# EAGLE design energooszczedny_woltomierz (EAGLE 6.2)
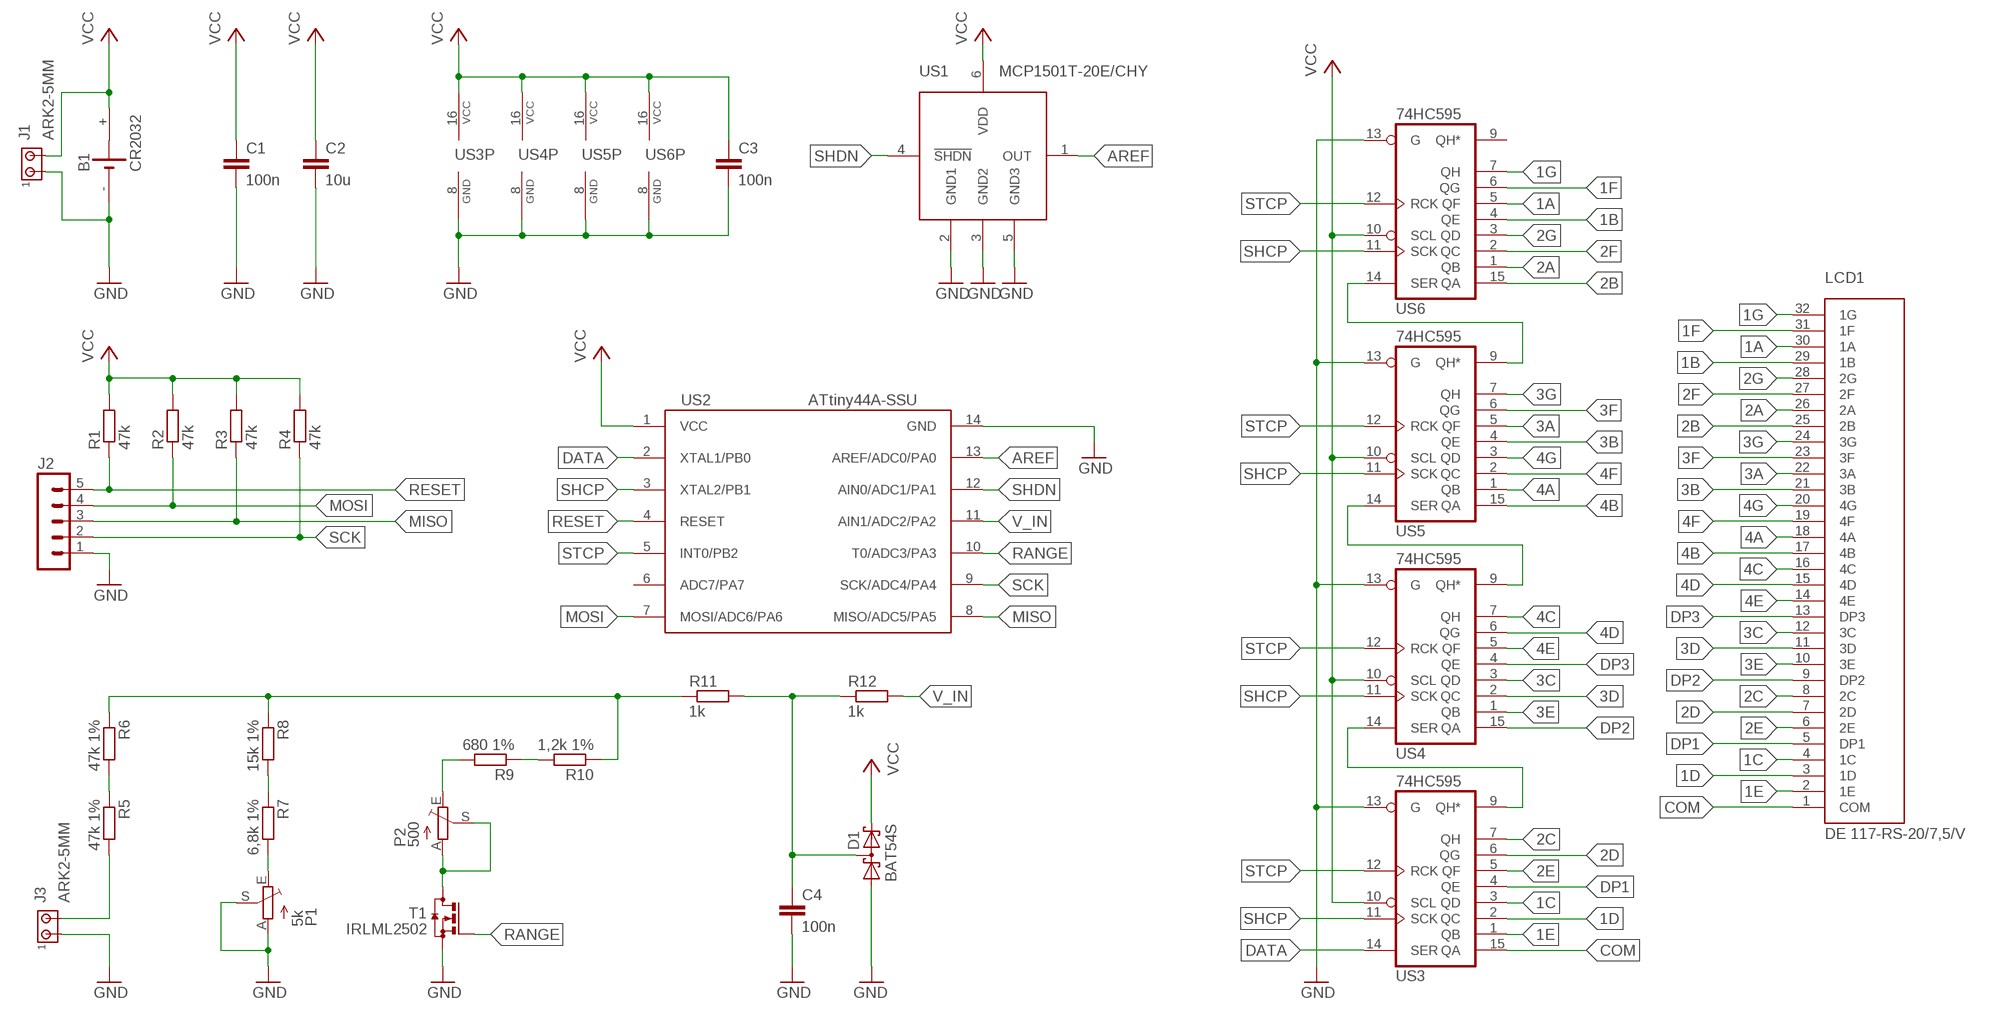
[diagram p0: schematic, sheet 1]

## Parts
B1  CR2032  BAT_20/16_XX  [BAT_CR2032]
C1  100n  C-EUC0805  [C0805]
C2  10u  C-EUC0805  [C0805]
C3  100n  C-EUC0805  [C0805]
C4  100n  C-EUC0805  [C0805]
D1  BAT54S  [SOT23]
J1  ARK2-5MM  [2PIN-5MM]
J2  MA05-1  [MA05-1]
J3  ARK2-5MM  [2PIN-5MM]
LCD1  DE 117-RS-20/7,5/V  LCD_DE117  [DE117]
P1  5k  TRIM_EU-CA6V  [CA6V]
P2  500  TRIM_EU-CA6V  [CA6V]
R1  47k  R-EU_R0805  [R0805]
R2  47k  R-EU_R0805  [R0805]
R3  47k  R-EU_R0805  [R0805]
R4  47k  R-EU_R0805  [R0805]
R5  47k 1%  R-EU_R0805  [R0805]
R6  47k 1%  R-EU_R0805  [R0805]
R7  6,8k 1%  R-EU_R0805  [R0805]
R8  15k 1%  R-EU_R0805  [R0805]
R9  680 1%  R-EU_R0805  [R0805]
R10  1,2k 1%  R-EU_R0805  [R0805]
R11  1k  R-EU_R0805  [R0805]
R12  1k  R-EU_R0805  [R0805]
T1  IRLML2502  BSS123  [SOT23]
US1  MCP1501T-20E/CHY  MCP1501  [SOT23-6]
US2  ATtiny44A-SSU  ATTINY24/44/84-SSU  [SOIC14]
US3  74HC595  74LS595D  [SO16]
US4  74HC595  74LS595D  [SO16]
US5  74HC595  74LS595D  [SO16]
US6  74HC595  74LS595D  [SO16]

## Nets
1A: LCD1.30(1A) US6.5(QF)
1B: LCD1.29(1B) US6.4(QE)
1C: LCD1.4(1C) US3.3(QD)
1D: LCD1.3(1D) US3.2(QC)
1E: LCD1.2(1E) US3.1(QB)
1F: LCD1.31(1F) US6.6(QG)
1G: LCD1.32(1G) US6.7(QH)
2A: LCD1.26(2A) US6.1(QB)
2B: LCD1.25(2B) US6.15(QA)
2C: LCD1.8(2C) US3.7(QH)
2D: LCD1.7(2D) US3.6(QG)
2E: LCD1.6(2E) US3.5(QF)
2F: LCD1.27(2F) US6.2(QC)
2G: LCD1.28(2G) US6.3(QD)
3A: LCD1.22(3A) US5.5(QF)
3B: LCD1.21(3B) US5.4(QE)
3C: LCD1.12(3C) US4.3(QD)
3D: LCD1.11(3D) US4.2(QC)
3E: LCD1.10(3E) US4.1(QB)
3F: LCD1.23(3F) US5.6(QG)
3G: LCD1.24(3G) US5.7(QH)
4A: LCD1.18(4A) US5.1(QB)
4B: LCD1.17(4B) US5.15(QA)
4C: LCD1.16(4C) US4.7(QH)
4D: LCD1.15(4D) US4.6(QG)
4E: LCD1.14(4E) US4.5(QF)
4F: LCD1.19(4F) US5.2(QC)
4G: LCD1.20(4G) US5.3(QD)
AREF: US1.1(OUT) US2.13(AREF/ADC0/PA0)
COM: LCD1.1(COM) US3.15(QA)
DATA: US2.2(XTAL1/PB0) US3.14(SER)
DP1: LCD1.5(DP1) US3.4(QE)
DP2: LCD1.9(DP2) US4.15(QA)
DP3: LCD1.13(DP3) US4.4(QE)
GND: B1.- C1.2 C2.2 C3.2 C4.2 D1.1(A1) J1.P$1 J2.1 J3.P$1 P1.A P1.S T1.2(S) US1.2(GND1) US1.3(GND2) US1.5(GND3) US2.14(GND) US3.8(GND) US3.13(G) US4.8(GND) US4.13(G) US5.8(GND) US5.13(G) US6.8(GND) US6.13(G)
MISO: J2.3 R3.1 US2.8(MISO/ADC5/PA5)
MOSI: J2.4 R2.1 US2.7(MOSI/ADC6/PA6)
N$1: J3.P$2 R5.2
N$2: R5.1 R6.2
N$3: R6.1 R8.1 R10.1 R11.1
N$4: C4.1 D1.3(C1A2) R11.2 R12.1
N$5: P2.A P2.S T1.3(D)
N$6: R7.1 R8.2
N$7: R9.1 R10.2
N$8: P1.E R7.2
N$9: P2.E R9.2
N$33: US3.9(QH*) US4.14(SER)
N$34: US4.9(QH*) US5.14(SER)
N$35: US5.9(QH*) US6.14(SER)
RANGE: T1.1(G) US2.10(T0/ADC3/PA3)
RESET: J2.5 R1.1 US2.4(RESET)
SCK: J2.2 R4.1 US2.9(SCK/ADC4/PA4)
SHCP: US2.3(XTAL2/PB1) US3.11(SCK) US4.11(SCK) US5.11(SCK) US6.11(SCK)
SHDN: US1.4(!SHDN) US2.12(AIN0/ADC1/PA1)
STCP: US2.5(INT0/PB2) US3.12(RCK) US4.12(RCK) US5.12(RCK) US6.12(RCK)
V_IN: R12.2 US2.11(AIN1/ADC2/PA2)
VCC: B1.+ C1.1 C2.1 C3.1 D1.2(C2) J1.P$2 R1.2 R2.2 R3.2 R4.2 US1.6(VDD) US2.1(VCC) US3.10(SCL) US3.16(VCC) US4.10(SCL) US4.16(VCC) US5.10(SCL) US5.16(VCC) US6.10(SCL) US6.16(VCC)
Unconnected: US2.6(ADC7/PA7) US6.9(QH*)

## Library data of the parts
B1 = inne_futrzak:BAT_20/16_XX
C1-C4 = rcl:C-EU: CAPACITOR, European symbol
D1 = diode:BAT54S: Schottky Diodes Pin connection corrected 2011-05-04 Source: Fairchild .. BAT54.pdf
J1 J3 = zlacza_futrzak:ARK2: ARK 2
J2 = zlacza_futrzak:MA05-1: PIN HEADER; OC_FARNELL: unknown; OC_NEWARK: unknown
LCD1 = inne_futrzak:LCD_DE117
P1 P2 = pot:TRIM_EU-: POTENTIOMETER
R1-R12 = rcl:R-EU_: RESISTOR, European symbol
T1 = transistor-small-signal:BSS123: N-CHANNEL MOS FET
US1 = scalaki_futrzak:MCP1501
US2 = scalaki_futrzak:ATTINY24/44/84
US3-US6 = scalaki_futrzak:74*595: 8-bit SHIFT REGISTER, output latch

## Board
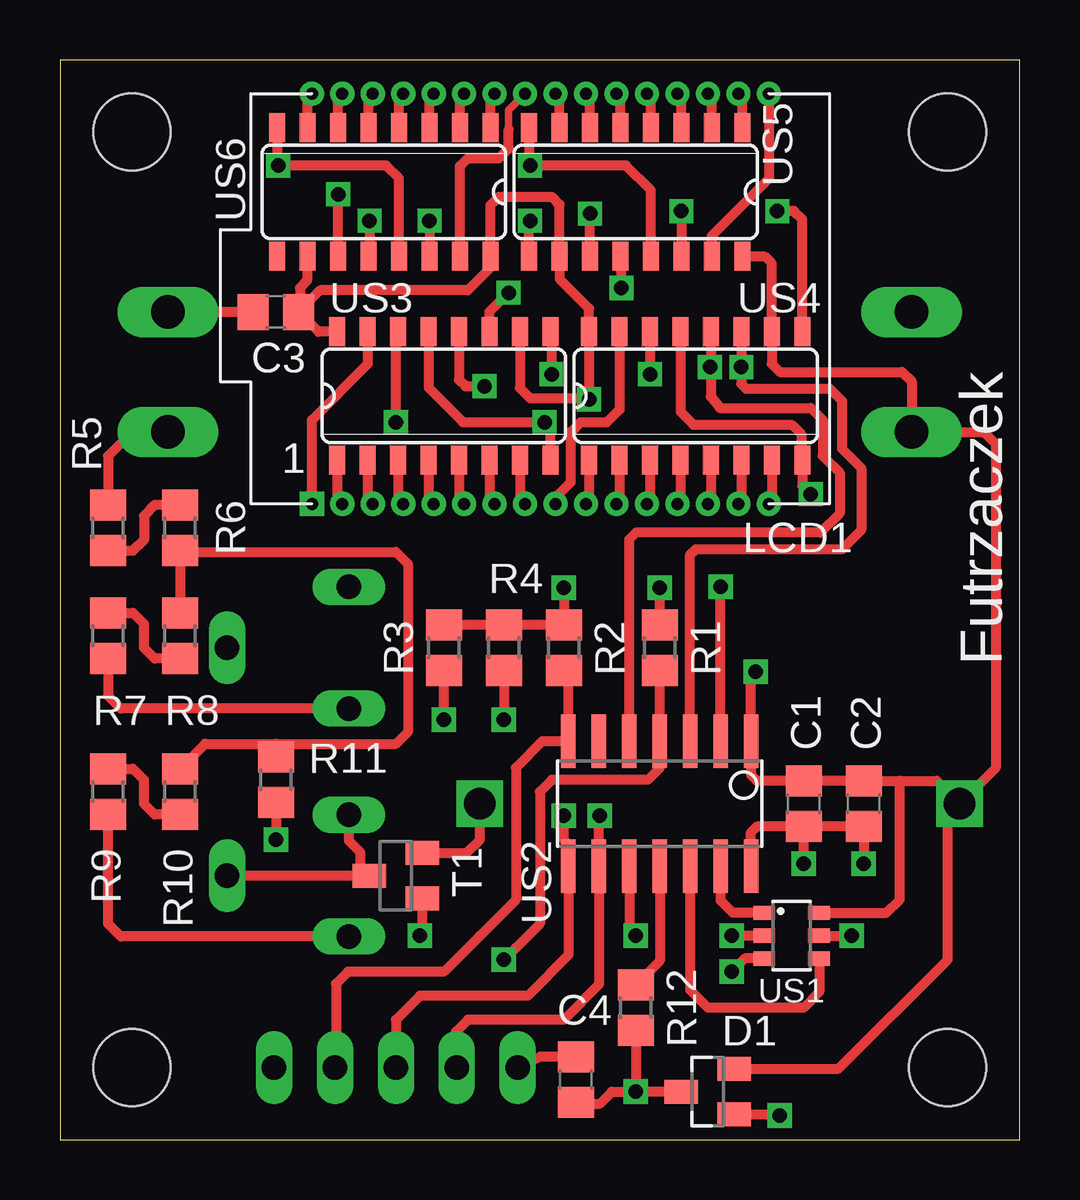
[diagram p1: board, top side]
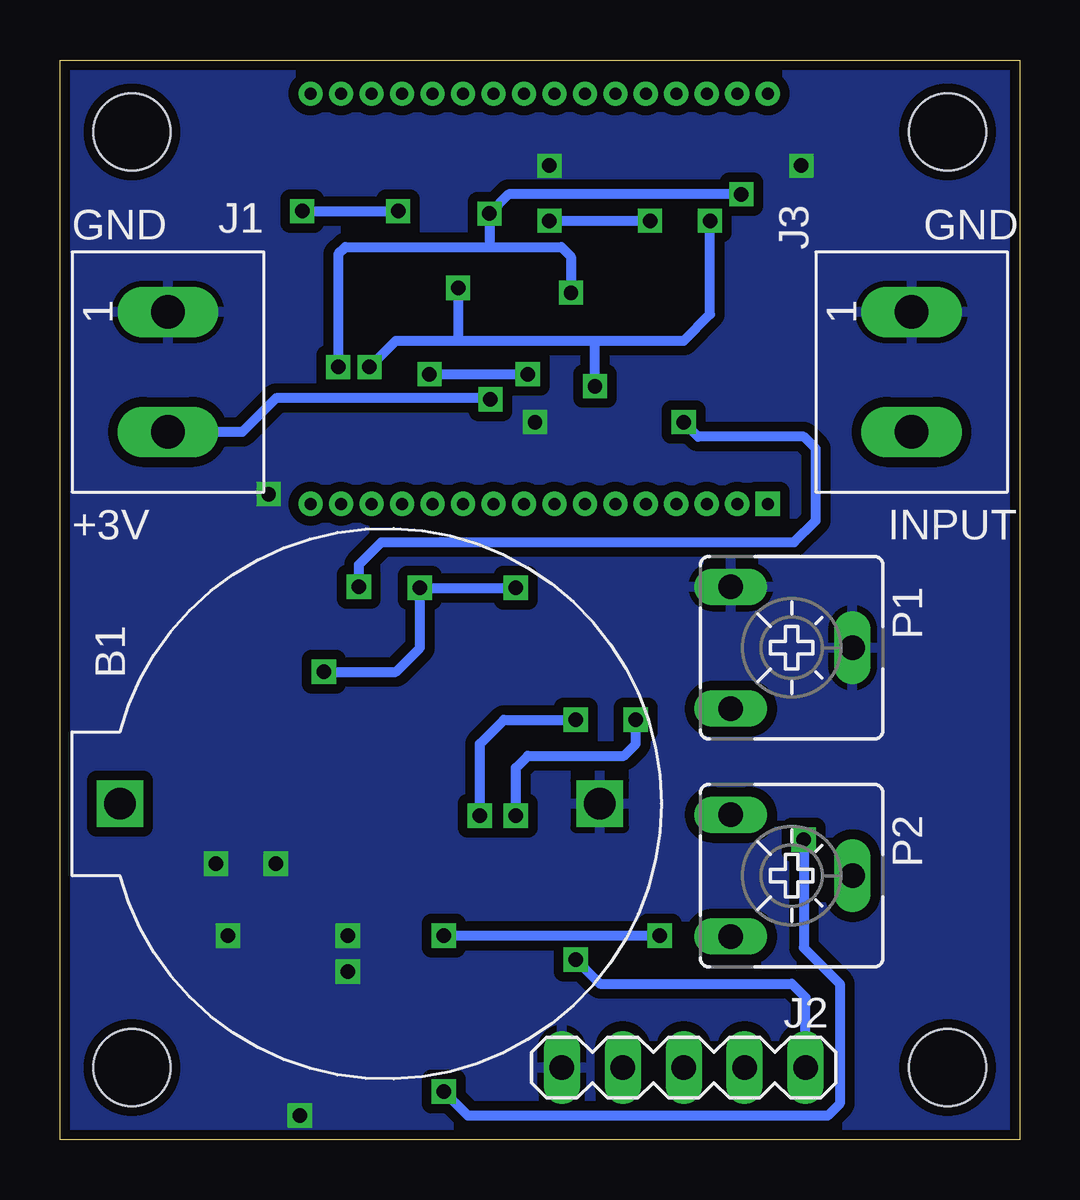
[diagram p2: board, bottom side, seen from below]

Size 40 x 45 mm. Coordinates in mm from the lower left corner, seen from the top.
Outline: 0,0 40,0 40,45 0,45 0,0
Copper layers (1*16): Top 0.035mm / dielectric 1.5mm / Bottom 0.035mm
Design rules: minimum track width 10mil, minimum drill 4mil, track to track 8mil, track to pad 8mil, pad to pad 8mil, via to via 8mil, smd to smd 8mil, copper to edge 15mil, drill to drill 8mil, minimum pad ring 10mil, minimum via ring 8mil, stop-mask expansion 4mil, vias tented up to drill 0mil, thermal gap 10mil
Holes 3.2 mm at 3,3 3,42 37,42 37,3

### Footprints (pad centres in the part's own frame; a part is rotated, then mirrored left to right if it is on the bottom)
BAT_CR2032 = drill 1.3 square: + 12,0; - -8,0
C0805 = smd 1.3 x 1.5: 1 -0.95,0; 2 0.95,0
SOT23 = smd 1 x 1.4: 1 -0.95,-1.1; 2 0.95,-1.1; 3 0,1.1
2PIN-5MM = drill 1.4 long: P$1 -2.5,0; P$2 2.5,0
MA05-1 = drill 1.016 long: 1 -5.08,0; 2 -2.54,0; 3 0,0; 4 2.54,0; 5 5.08,0
DE117 = drill 0.5 square: 1 0,0 | drill 0.5: 2 1.27,0; 3 2.54,0; 4 3.81,0; 5 5.08,0; 6 6.35,0; 7 7.62,0; 8 8.89,0; 9 10.16,0; 10 11.43,0; 11 12.7,0; 12 13.97,0; 13 15.24,0; 14 16.51,0; 15 17.78,0; 16 19.05,0; 17 19.05,17.1; 18 17.78,17.1; 19 16.51,17.1; 20 15.24,17.1; 21 13.97,17.1; 22 12.7,17.1; 23 11.43,17.1; 24 10.16,17.1; 25 8.89,17.1; 26 7.62,17.1; 27 6.35,17.1; 28 5.08,17.1; 29 3.81,17.1; 30 2.54,17.1; 31 1.27,17.1; 32 0,17.1
CA6V = drill 1.016 long: A -2.54,-2.54; E 2.54,-2.54; S 0,2.54
R0805 = smd 1.3 x 1.5: 1 -0.95,0; 2 0.95,0
SOT23-6 = smd 0.6 x 0.9: 1 -0.95,-1.15; 2 0,-1.15; 3 0.95,-1.15; 4 0.95,1.15; 5 0,1.15; 6 -0.95,1.15
SOIC14 = smd 0.61 x 2.21: 1 -3.81,-2.603; 2 -2.54,-2.603; 3 -1.27,-2.603; 4 0,-2.603; 5 1.27,-2.603; 6 2.54,-2.603; 7 3.81,-2.603; 8 3.81,2.603; 9 2.54,2.603; 10 1.27,2.603; 11 0,2.603; 12 -1.27,2.603; 13 -2.54,2.603; 14 -3.81,2.603
SO16 = smd 0.66 x 1.2: 1 -4.445,-2.673; 2 -3.175,-2.673; 3 -1.905,-2.673; 4 -0.635,-2.673; 5 0.635,-2.673; 6 1.905,-2.673; 7 3.175,-2.673; 8 4.445,-2.673; 9 4.445,2.673; 10 3.175,2.673; 11 1.905,2.673; 12 0.635,2.673; 13 -0.635,2.673; 14 -1.905,2.673; 15 -3.175,2.673; 16 -4.445,2.673

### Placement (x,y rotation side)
B1  25.5,14 180 bottom
C1  31,14 270 top
C2  33.5,14 270 top
C3  9,34.5 180 top
C4  21.5,2.5 90 top
D1  27,2 90 top
J1  35.5,32 270 bottom
J2  14,3 0 bottom
J3  4.5,32 270 bottom
LCD1  10.5,26.5 0 top
P1  9.5,20.5 270 bottom
P2  9.5,11 270 bottom
R1  25,20.5 90 top
R2  21,20.5 90 top
R3  16,20.5 90 top
R4  18.5,20.5 90 top
R5  2,25.5 90 top
R6  5,25.5 90 top
R7  2,21 270 top
R8  5,21 270 top
R9  2,14.5 270 top
R10  5,14.5 270 top
R11  9,15 270 top
R12  24,5.5 90 top
T1  14,11 90 top
US1  30.5,8.5 270 top
US2  25,14 180 top
US3  16,31 0 top
US4  26.5,31 0 top
US5  24,39.5 180 top
US6  13.5,39.5 180 top

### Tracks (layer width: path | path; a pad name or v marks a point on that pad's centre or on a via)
1A
  Top 0.406: US6.5 12.87,43.42 LCD1.30
1B
  Top 0.406: US6.4 14.13,43.42 LCD1.29
1C
  Top 0.406: US3.3 14.1,26.71 LCD1.4
1D
  Top 0.406: US3.2 12.82,26.71 LCD1.3
1E
  Top 0.406: US3.1 11.55,26.71 LCD1.2
1F
  Top 0.406: US6.6 11.6,43.42 LCD1.31
1G
  Top 0.406: US6.7 10.32,43.42 LCD1.32
2A
  Top 0.406: US6.1 17.95,43.42 LCD1.26
2B
  Top 0.305: 18.7,42.1 18.7,42.91 LCD1.25
  Top 0.406: US6.15 16.68,40.58 17,40.9 18.3,40.9 18.7,41.3 18.7,42.1
2C
  Top 0.406: US3.7 19.18,26.71 LCD1.8
2D
  Top 0.406: US3.6 17.91,26.71 LCD1.7
2E
  Top 0.406: US3.5 16.64,26.71 LCD1.6
2F
  Top 0.406: US6.2 16.68,43.42 LCD1.27
2G
  Top 0.406: US6.3 15.4,43.42 LCD1.28
3A
  Top 0.406: US5.5 23.36,43.44 LCD1.22
3B
  Top 0.406: US5.4 24.64,43.44 LCD1.21
3C
  Top 0.406: US4.3 24.59,26.62 LCD1.12
3D
  Top 0.406: US4.2 23.32,26.62 LCD1.11
3E
  Top 0.406: US4.1 22.05,26.62 LCD1.10
3F
  Top 0.406: US5.6 22.09,43.44 LCD1.23
3G
  Top 0.406: US5.7 20.82,43.44 LCD1.24
4A
  Top 0.406: US5.1 28.45,43.44 LCD1.18
4B
  Top 0.406: LCD1.17 29.55,40.05 27.18,37.67 US5.15
4C
  Top 0.406: US4.7 29.68,26.62 LCD1.16
4D
  Top 0.406: US4.6 28.41,26.62 LCD1.15
4E
  Top 0.406: US4.5 27.14,26.62 LCD1.14
4F
  Top 0.406: US5.2 27.18,43.44 LCD1.19
4G
  Top 0.406: US5.3 25.91,43.44 LCD1.20
AREF
  Top 0.406: US1.1 28.05,9.45 28,9.5 27.54,9.96 US2.13
COM
  Top 0.406: LCD1.1 10.5,30 12.82,32.33 US3.15
DATA  (via drill 0.6)
  Top 0.406: US2.2 v27.54,23.04 | v14,29.9 14,33.58 US3.14
  Bottom 0.406: v27.54,23.04 27.54,23.96 26.6,24.9 9.4,24.9 8.5,25.8 8.5,28.8 9,29.3 13.4,29.3 v14,29.9
DP1
  Top 0.406: US3.4 15.37,26.71 LCD1.5
DP2
  Top 0.406: US4.15 23.32,30.43 22.8,29.9 21.7,29.9 21.3,29.5 21.3,27.4 20.66,26.76 LCD1.9
DP3
  Top 0.406: US4.4 25.86,26.62 LCD1.13
GND  (via drill 0.6)
  Top 0.406: T1.2 16.95,11.95 17.5,12.5 B1.- | C1.2 C2.2 v33.5,11.5 | C1.2 29.05,13.05 28.81,12.81 US2.14 | v31,11.5 C1.2 | C4.2 20.03,3.45 J2.1 | D1.1 29.95,1.05 v30,1 | C3.2 J3.P$1 | 9.05,42.45 US6.8 9.05,40.65 v9.1,40.6 13.6,40.6 14.13,40.06 US6.13 | US5.8 19.55,40.65 v19.6,40.6 23.6,40.6 24.64,39.56 US5.13 | US3.8 20.45,29.66 v20.2,29.9 16.8,29.9 15.37,31.34 US3.13 | v31.3,26.9 30.95,27.25 US4.8 30.9,28.37 30.9,29.4 30.5,29.8 26.4,29.8 25.86,30.34 US4.13 | US1.2 v28,8.5 | v28,7 28.35,7.35 28.55,7.55 US1.3 | US1.5 v33,8.5
  pour Bottom (isolate 0.406): 0,45 40,45 40,0 0,0
MISO  (via drill 0.6)
  Top 0.406: J2.3 14,5 15,6 19.5,6 21.19,7.69 US2.8 21.19,12.31 21,12.5 v21,13.5 | v16,17.5 R3.1
  Bottom 0.406: v21,13.5 21,15.5 20.5,16 16.5,16 16,16.5 v16,17.5
MOSI
  Top 0.406: J2.4 11.5,2.54 11.5,6.5 12,7 16,7 17.5,8.5 19,10 19,15.5 20.1,16.6 US2.7 21.19,19.36 R2.1
N$1
  Top 0.406: J3.P$2 3,29.5 2,28.5 R5.2
N$2
  Top 0.406: R5.1 3.05,24.55 3.5,25 3.5,26 3.95,26.45 R6.2
N$3
  Top 0.406: R8.1 R6.1 5.05,24.5 14,24.5 14.5,24 14.5,17 14,16.5 9,16.5 | 9,16.5 6.05,16.5 R10.1 | R11.1 9,16.5
N$4  (via drill 0.6)
  Top 0.406: R12.1 v24,2 | C4.1 21.55,1.5 22.5,1.5 23,2 v24,2 | R11.2 v9,12.5 | D1.3 v24,2
  Bottom 0.406: v9,12.5 9,8 7.5,6.5 7.5,1.5 8,1 23,1 v24,2
N$5
  Top 0.406: P2.S T1.3 12.5,11.4 12.5,12 12.04,12.46 P2.A
N$6
  Top 0.406: R7.1 3.05,21.95 3.5,21.5 3.5,20.5 3.95,20.05 R8.2
N$7
  Top 0.406: R9.1 3.05,15.45 3.5,15 3.5,14 3.95,13.55 R10.2
N$8
  Top 0.406: R7.2 2,18.5 2.54,17.96 P1.E
N$9
  Top 0.406: P2.E 2.54,8.46 2,9 R9.2
N$33  (via drill 0.6)
  Top 0.406: US4.14 v24.59,31.91 v24.6,31.9 | v20.5,31.9 20.5,33.62 US3.9
  Bottom 0.406: v24.6,31.9 v20.5,31.9
N$34  (via drill 0.6)
  Top 0.406: US4.9 30.95,38.35 30.6,38.7 v29.9,38.7 | v25.9,38.7 US5.14
  Bottom 0.406: v29.9,38.7 v25.9,38.7
N$35  (via drill 0.6)
  Top 0.406: US5.9 19.55,38.26 v19.6,38.3 | v15.4,38.3 US6.14
  Bottom 0.406: v19.6,38.3 v15.4,38.3
RANGE  (via drill 0.6)
  Top 0.406: T1.1 15.1,8.6 v15,8.5 | US2.10 23.73,8.77 v24,8.5
  Bottom 0.406: v15,8.5 v24,8.5
RESET  (via drill 0.6)
  Top 0.406: R1.1 US2.4 25,15.5 24.5,15 20.5,15 20,14.5 20,9 19,8 v18.5,7.5
  Bottom 0.406: v18.5,7.5 17.5,6.5 9.5,6.5 8.92,5.92 J2.5
SCK  (via drill 0.6)
  Top 0.406: J2.2 16.5,2.54 16.5,4.5 17,5 21,5 22.46,6.46 US2.9 22.46,13.46 v22.5,13.5 | R4.1 v18.5,17.5
  Bottom 0.406: v22.5,13.5 22.5,16.5 21.5,17.5 v18.5,17.5
SHCP  (via drill 0.6)
  Top 0.406: US2.3 26.27,24.37 26.5,24.6 32.6,24.6 33.4,25.4 33.4,28 32.6,28.8 32.6,30.8 32.1,31.3 28.6,31.3 28.41,31.5 v28.41,32.2 | US4.11 v28.41,32.2 | US6.11 v11.6,39.4 | US3.11 17.91,34.51 v18.7,35.3 | US5.11 v22.09,38.59 v22.1,38.6 | v28.4,32.2 v28.41,32.2
  Bottom 0.406: 22.2,37.2 28.1,37.2 28.4,36.9 v28.4,32.2 | 22.2,37.2 22.1,37.3 v22.1,38.6 21.3,39.4 v11.6,39.4 | 22.2,37.2 19.1,37.2 18.7,36.8 v18.7,35.3
SHDN
  Top 0.406: US1.4 31.65,6.15 31,5.5 27,5.5 26.5,6 26.27,6.23 US2.12
STCP  (via drill 0.6)
  Top 0.406: US2.5 23.73,25.03 24,25.3 31.7,25.3 32.5,26.1 32.5,27.8 31.8,28.5 31.8,30 31.3,30.5 27.5,30.5 27.14,30.96 27.14,32.2 | US4.12 27.14,32.2 | v12.9,38.3 12.9,36.79 US6.12 | US3.12 16.64,31.66 16.9,31.4 v17.7,31.4 | v27.1,32.2 27.14,32.2 | v23.4,35.5 23.4,36.79 US5.12
  Bottom 0.406: 23.4,33.3 26,33.3 v27.1,32.2 | 23.4,33.3 17.7,33.3 | 17.7,33.3 14,33.3 12.9,34.4 v12.9,38.3 | v17.7,31.4 17.7,33.3 | v23.4,35.5 23.4,33.3
V_IN
  Top 0.406: US2.11 25,7.45 R12.2
VCC  (via drill 0.6)
  Top 0.406: R1.2 v25,23 | v21,23 R2.2 R4.2 R3.2 | v29,19.5 28.81,19.31 US2.1 28.81,15.19 29.05,14.95 C1.1 C2.1 35,14.95 | 35,14.95 36.55,14.95 B1.+ | B1.+ 39,15.5 39,29 38.5,29.5 J1.P$2 35.5,31.6 35.1,32 30,32 29.68,32.33 US4.10 29.68,36.52 29.4,36.8 28.47,36.8 US5.16 | B1.+ 37,13.5 37,9.5 37,7.5 32.45,2.95 D1.2 | US3.10 19.18,31.32 19.5,31 19.6,30.9 22.01,30.9 v22.05,30.86 | v22.05,30.86 US4.16 22.05,34.65 20.82,35.88 US5.10 20.82,38.98 20.5,39.3 18.3,39.3 17.95,38.95 US6.16 17.95,36.34 17,35.4 11.6,35.4 10.85,35.4 C3.1 | US6.10 10.3,36.8 10.3,35.8 10,35.5 10,34.55 C3.1 | 22,30.8 v22.05,30.86 | US3.16 10.78,33.67 C3.1 | US1.6 34.45,9.45 35,10 35,14.95
  Bottom 0.406: v21,23 v25,23 25,20.5 26,19.5 v29,19.5 | v22.05,30.86 22.1,30.9 31,30.9 32.4,29.5 J1.P$2

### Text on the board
tPlace: Futrzaczek
bPlace: GND | GND | INPUT | +3V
